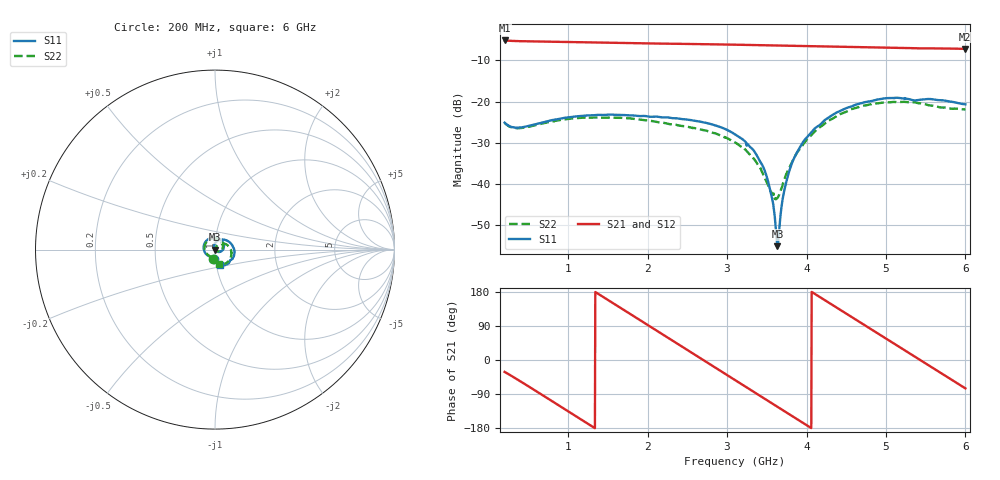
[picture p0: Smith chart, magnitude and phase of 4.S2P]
!Agilent Technologies,E5071C,MY46316741,A.11.02
!Date: Fri Apr 15 16:19:56 2022
!Data & Calibration Information:
!Freq	S11:SOLT2(ON)	S21:SOLT2(ON)	S12:SOLT2(ON)	S22:SOLT2(ON)
!PortZ  Port1:50+j0  Port2:50+j0
!Above PortZ is port z conversion or system Z0 setting when saving the data.
!When reading, reference impedance value at option line is always used.
# Hz S dB R 50
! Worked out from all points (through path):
!   1200 points, 200 MHz to 6 GHz, reference 50 ohm
!   highest |S21| = -5.15 dB at 200 MHz (marker M1); lowest = -7.2 dB at 5.99 GHz (marker M2)
!   group delay of S21, straight-line fit = 367 ps
!   lowest |S11| = -55.1 dB at 3.635 GHz (marker M3), VSWR 1.00, Z = 49.9 - j0.104 ohm
!   |S11| at or under -10 dB: start of sweep to end of sweep
!   |S22| runs from -43.7 to -20.1 dB; largest |S21 - S12| = 0.0016
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2e8  -25.13 -95.7  -5.15 -31.4  -5.16 -31.4  -25.17 -103.3
6.837364e8  -25.04 -155.2  -5.45 -93.6  -5.45 -93.6  -25.32 -166.7
1.167473e9  -23.50 154.7  -5.62 -157.6  -5.62 -157.5  -23.96 141.0
1.573812e9  -23.21 118.2  -5.76 148.8  -5.76 148.8  -23.94 102.6
1.864053e9  -23.46 94.2  -5.84 110.5  -5.85 110.6  -24.29 76.1
2.134946e9  -23.70 73.7  -5.91 74.8  -5.91 74.8  -25.03 54.2
2.633194e9  -24.77 33.7  -6.04 8.9  -6.04 8.9  -26.62 18.7
2.86055e9  -25.84 14.0  -6.11 -21.2  -6.11 -21.2  -27.79 2.0
3.102419e9  -28.00 -8.5  -6.18 -53.2  -6.19 -53.1  -29.93 -15.7
3.329775e9  -31.74 -32.0  -6.26 -83.3  -6.26 -83.2  -33.70 -29.8
3.460384e9  -36.10 -48.0  -6.31 -100.5  -6.30 -100.4  -37.96 -29.4
3.557131e9  -42.71 -67.7  -6.34 -113.3  -6.34 -113.2  -42.08 -10.9
3.634529e9  -55.13 -143.3  -6.36 -123.5  -6.36 -123.5  -43.42 32.1
3.653878e9  -51.71 166.2  -6.37 -126.1  -6.37 -126.0  -42.73 40.3
3.716764e9  -41.93 130.4  -6.39 -134.4  -6.39 -134.3  -39.16 58.9
3.798999e9  -35.90 113.4  -6.43 -145.3  -6.43 -145.2  -35.48 65.2
4.069892e9  -27.23 80.6  -6.53 179.0  -6.53 179.1  -27.97 52.5
4.58749e9  -21.01 29.6  -6.70 110.8  -6.70 110.9  -21.72 9.8
5.037364e9  -19.15 -10.5  -6.88 51.6  -6.88 51.7  -20.19 -28.2
5.501751e9  -19.41 -42.3  -7.08 -9.2  -7.08 -9.1  -20.70 -59.4
5.990325e9  -20.64 -70.6  -7.20 -73.6  -7.20 -73.6  -21.91 -75.0
6e9  -20.67 -70.9  -7.19 -74.9  -7.20 -74.8  -21.92 -75.2
